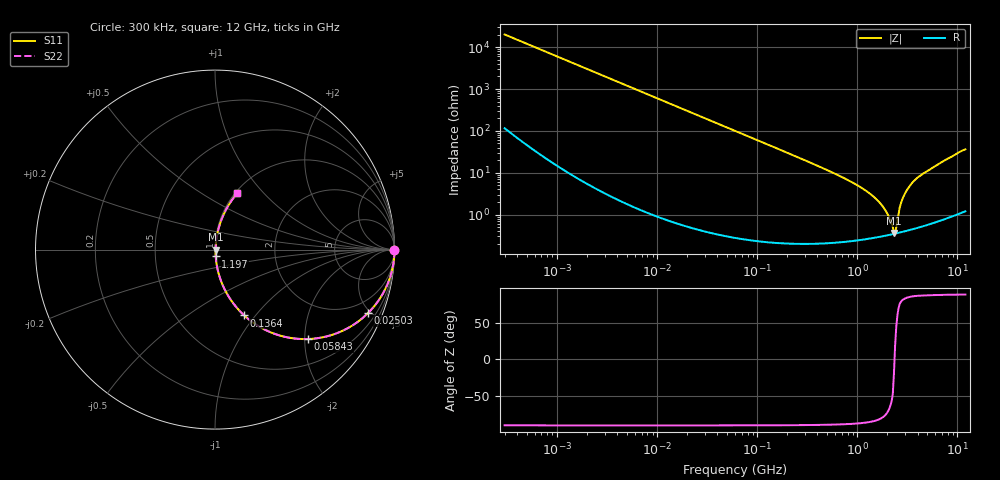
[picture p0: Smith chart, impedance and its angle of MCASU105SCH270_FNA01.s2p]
! MCASU105SCH270_FNA01  S-PARAMETER MODEL  ( General Type )
! Model Generated by TAIYO YUDEN Corporation (http://www.ty-top.com)
! Version 1.0
! TAIYO YUDEN Control No. 130207
! Copyright(c) 2013 TAIYO YUDEN CO.,LTD. All Rights Reserved.
! Product Description (link to TY-COMPAS)
! https://ds.yuden.co.jp/TYCOMPAS/or/detail?pn=MCASU105SCH270JFNA01&u=M
! Products Name : Multilayer Ceramic Capacitors
! Characteristics :
!  Capacitance : 27 pF , Rated Voltage : 50V , TCC : CH / C0H
!  Case Size : 1.0 x 0.5 / 0.039 x 0.02 [mm/inch] , Thickness : 0.5 / 0.02 [mm/inch]
!  (Conditions: Temperature = 25 degC , DC Bias Current/Voltage = 0A / 0V)
! External Node Assignments :
!  1  o---| |---o  2
! GND o---------o GND
! Frequency Range : 300000Hz  -  12GHz  [ 401 STEP ]
# MHz S RI R 50
! Freq[MHz].  S11 Real  S11 Imag  S21 Real  S21 Imag  S12 Real  S12 Imag  S22 Real  S22 Imag
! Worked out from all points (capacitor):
!   401 points, 300 kHz to 12 GHz, reference 50 ohm
!   read as one part in series: C = 26.4 pF near 316.3 kHz
!   lowest |Z| = 365 mohm at 2.322 GHz (marker M1)
!   series resonance near 2.353 GHz, so ESL is about 170 pH
!   S11 on the Smith chart (normalised r, x): 300 kHz: open; 25.03 MHz: 1.01, -4.82; 58.43 MHz: 1.01, -2.06; 136.4 MHz: 1.00, -0.88; 1.197 GHz: 1.01, -0.08; 12 GHz: 1.02, +0.72
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0.3  0.9999 -0.00497  5.33e-05 0.00497  5.33e-05 0.00497  0.9999 -0.00497
1.769972  0.9991 -0.0293  0.000914 0.0293  0.000914 0.0293  0.9991 -0.0293
10.44266  0.9707 -0.1679  0.0293 0.1679  0.0293 0.1679  0.9707 -0.1679
25.03118  0.8527 -0.3535  0.1473 0.3535  0.1473 0.3535  0.8527 -0.3535
58.43137  0.5158 -0.4984  0.4842 0.4984  0.4842 0.4984  0.5158 -0.4984
60  0.5026 -0.4986  0.4974 0.4986  0.4974 0.4986  0.5026 -0.4986
136.3989  0.163 -0.3669  0.837 0.3669  0.837 0.3669  0.163 -0.3669
353.9943  0.0289 -0.1617  0.9711 0.1617  0.9711 0.1617  0.0289 -0.1617
743.2595  0.00758 -0.0729  0.9924 0.0729  0.9924 0.0729  0.00758 -0.0729
1197.383  0.00401 -0.038  0.996 0.038  0.996 0.038  0.00401 -0.038
1689.663  0.00329 -0.0184  0.9967 0.0184  0.9967 0.0184  0.00329 -0.0184
1878.541  0.00327 -0.0129  0.9967 0.0129  0.9967 0.0129  0.00327 -0.0129
2088.533  0.00332 -0.00762  0.9967 0.00762  0.9967 0.00762  0.00332 -0.00762
2261.293  0.00342 -0.0036  0.9966 0.0036  0.9966 0.0036  0.00342 -0.0036
2321.999  0.00345 -0.00115  0.9965 0.00115  0.9965 0.00115  0.00345 -0.00115
2448.343  0.00356 0.00348  0.9964 -0.00348  0.9964 -0.00348  0.00356 0.00348
2722.03  0.0041 0.018  0.9959 -0.018  0.9959 -0.018  0.0041 0.018
2870.14  0.00454 0.0254  0.9955 -0.0254  0.9955 -0.0254  0.00454 0.0254
3190.978  0.00583 0.0409  0.9942 -0.0409  0.9942 -0.0409  0.00583 0.0409
3642.919  0.00834 0.0616  0.9917 -0.0616  0.9917 -0.0616  0.00834 0.0616
6354.153  0.0305 0.1517  0.9695 -0.1517  0.9695 -0.1517  0.0305 0.1517
12000  0.124 0.3134  0.876 -0.3134  0.876 -0.3134  0.124 0.3134
